{attribute 'qualified_only'}
{attribute 'strict'}
TYPE E_DirectControlState : 
(
	Ready := 0,
	WaitForActivationTime := 1,
	PerformTest := 2,
	WaitForExecution := 3,
	Operate := 4,
	WaitForChange := 5,
	MirrorBlockedCommand := 6
) ;
END_TYPE
